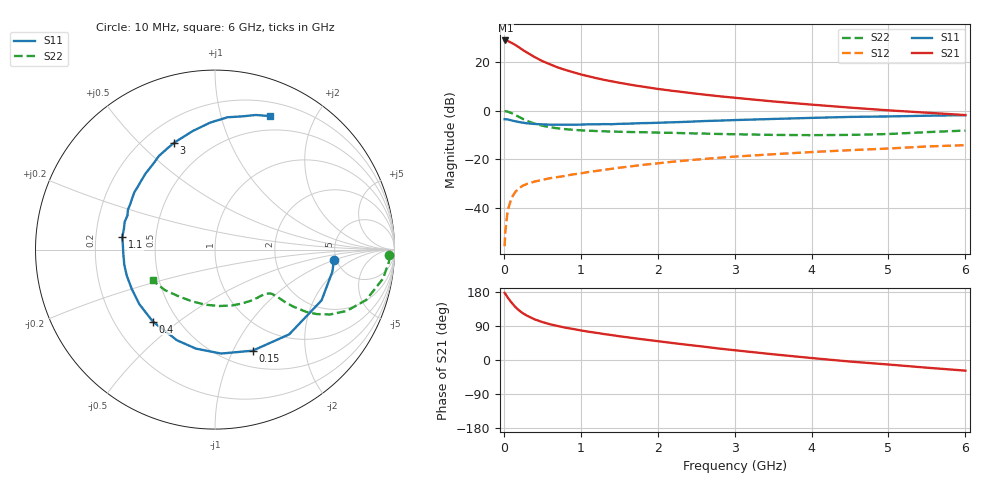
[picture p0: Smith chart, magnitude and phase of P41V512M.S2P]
! SIEMENS Small Signal Semiconductors
! BFP182
! Si NPN RF Bipolar Junction Transistor in SOT143
! VCE = 1.5 V  IC = 12 mA
! Common Emitter S-Parameters:  March  1996
# GHz  S  MA  R  50
!  f  S11  S21  S12  S22
! GHz  MAG  ANG  MAG  ANG  MAG  ANG  MAG  ANG
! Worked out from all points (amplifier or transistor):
!   36 points, 10 MHz to 6 GHz, reference 50 ohm
!   highest |S21| = 28.9 dB at 20 MHz (marker M1)
!   |S21| within 3 dB of that: start of sweep to 204.6 MHz
!   unconditionally stable (mu >= 1): 920 MHz to 5.47 GHz
!   at 250 MHz: K = 0.40, MSG = 27.9 dB, |S12| = -30.9 dB
!   at 1.4 GHz: K = 1.17, MAG = 15.6 dB, |S12| = -24.0 dB
!   at 6 GHz: K = 0.94, MSG = 6.2 dB, |S12| = -14.3 dB
!   S11 on the Smith chart (normalised r, x): 10 MHz: 4.74, -1.02; 150 MHz: 0.68, -1.20; 400 MHz: 0.36, -0.41; 1.1 GHz: 0.32, +0.06; 3 GHz: 0.32, +0.64; 6 GHz: 0.34, +1.44
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0.01  0.665 -5.2  27.73 177.1  0.0016 85.8  0.9714 -1.9
0.02  0.6655 -10.6  27.95 174.4  0.0033 76.7  0.9717 -4.0
0.05  0.6576 -25.5  27.29 165.0  0.0087 81.6  0.9498 -9.8
0.1  0.6276 -48.8  24.99 151.5  0.0158 68.1  0.8881 -18.4
0.15  0.601 -69.6  22.55 139.8  0.0211 60.3  0.8092 -25.0
0.2  0.5802 -86.6  20.02 130.5  0.0253 55.3  0.7359 -29.4
0.25  0.562 -100.8  17.65 123.0  0.0284 51.3  0.6704 -32.4
0.3  0.548 -112.7  15.77 117.1  0.0307 48.6  0.6162 -34.3
0.4  0.5298 -130.8  12.72 107.3  0.0344 46.0  0.5382 -36.1
0.5  0.5198 -144.2  10.5 100.2  0.0373 44.1  0.4884 -36.8
0.6  0.513 -154.6  9.017 94.4  0.0403 44.5  0.4542 -37.0
0.7  0.5126 -163.5  7.761 89.7  0.0426 45.0  0.4307 -37.2
0.8  0.5125 -170.4  6.905 85.3  0.0451 45.4  0.4139 -37.6
1  0.5138 177.4  5.574 78.1  0.0507 45.9  0.3924 -38.6
1.1  0.5214 172.2  5.101 74.7  0.0542 46.3  0.3851 -39.5
1.5  0.5332 155.6  3.75 62.7  0.0663 47.1  0.3667 -43.9
2.2  0.5743 132.2  2.548 44.6  0.0883 44.7  0.3471 -55.4
3  0.6371 111.1  1.84 25.8  0.1125 39.4  0.3254 -73.0
3.5  0.6723 100.6  1.545 15.1  0.1258 35.3  0.3152 -85.8
4.5  0.7406 84.6  1.153 -4.1  0.1527 27.5  0.3153 -114.0
5.5  0.7838 73.1  0.905 -20.3  0.1821 19.7  0.3594 -141.2
6  0.8041 67.7  0.809 -28.1  0.1936 14.7  0.3875 -153.7
